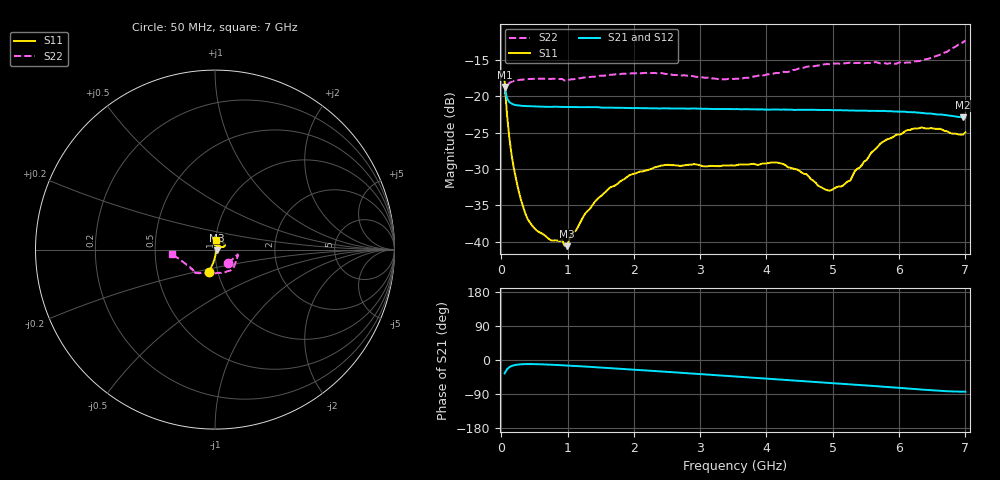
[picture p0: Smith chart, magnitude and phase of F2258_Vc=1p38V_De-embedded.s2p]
! Integrated Device Technology
! Corporate Headquarters
! 6024 Silver Creek Valley Road
! San Jose, CA 95138  USA
! Phone:  1-408-284-8200
! Toll Free:  1-800-223-1366
! Webpage:  http://www.idt.com/
! Timing and RF Division
! 515 Groton Road, Suite 102
! Westford, MA 01886-6024
! Device:  F2258
! Description: Voltage Variable RF Attenuator
! Frequency:  50.0 -  6000.00 MHz
! Package:  3x3 mm Thin QFN Plastic Package: 16 pin
! Ports:  2 RF, 2 DC
!  Pin  1  = NC
!  Pin  2  = NC
!  Pin  3  = RF2  = Port 2
!  Pin  4  = GND
!  Pin  5  = Vdd
!  Pin  6  = NC
!  Pin  7  = VCTRL
!  Pin  8  = NC
!  Pin  9  = GND
!  Pin 10  = RF1  = Port 1
!  Pin 11  = NC
!  Pin 12  = NC
!  Pin 13  = NC
!  Pin 14  = NC
!  Pin 15  = NC
!  Pin 16  = NC
! Vcntrl:  1.380 Volts
! Vdd:  +3.300 Volts
! Current:  1.166 mA
! Data:  The device was measured on a the F2258 evaluation board which has
!  individual transmission lines to the RF pins.  Data was collected
!  using a calibrated network analyzer.  The evaluation board was
!  de-embedded using a TRL calibration technique.
!  The reference plane is the edge of the package pin.
! Misc:  SN 10
!  Action Tracker AT0285
! Date Measured:  2014-12-10
! Date:  2016-01-13  MJV
! Note:
!  Integrated Device Technology supplies this data as a sample of measured
!  data at the package pin for this product.  Your particular data for this
!  product may vary.
!  Data was taken at 25 degrees C.
!  Integrated Device Technology reserves the right to change this data at anytime.
!Freq_(GHz)  S11M_(dB)  S11P_(deg)  S21M_(dB)  S21P_(deg)  S12M_(dB)  S12P_(deg)  S22M_(dB)  S22P_(deg)
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# GHz S dB R 50
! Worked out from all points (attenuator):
!   201 points, 50 MHz to 7 GHz, reference 50 ohm
!   highest |S21| = -18.72 dB at 50 MHz (marker M1); lowest = -22.9 dB at 6.965 GHz (marker M2)
!   lowest |S11| = -40.6 dB at 988.2 MHz (marker M3), VSWR 1.02, Z = 50.9 - j0.398 ohm
!   |S11| at or under -10 dB: start of sweep to end of sweep
!   |S22| runs from -19.7 to -12.3 dB; largest |S21 - S12| = 0.0006
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0.05  -17.93 -105.0  -18.72 -35.4  -18.73 -35.5  -19.68 -45.6
0.08475  -22.40 -97.9  -20.26 -24.7  -20.26 -24.7  -18.67 -22.8
0.15425  -28.01 -89.9  -21.01 -15.9  -21.03 -15.9  -18.01 -14.2
0.2585  -32.89 -79.7  -21.26 -11.9  -21.28 -11.9  -17.78 -12.0
0.36275  -36.12 -68.6  -21.35 -10.8  -21.36 -10.8  -17.67 -12.8
0.5365  -38.46 -49.0  -21.41 -11.0  -21.43 -11.0  -17.59 -15.5
0.98825  -40.60 -24.8  -21.48 -14.5  -21.50 -14.5  -17.80 -25.9
1.05775  -38.96 -16.3  -21.48 -15.2  -21.52 -15.2  -17.68 -27.3
1.2315  -36.65 -5.0  -21.49 -17.0  -21.50 -17.0  -17.45 -31.0
1.6485  -32.50 6.2  -21.57 -21.6  -21.59 -21.6  -17.06 -39.4
1.9265  -30.89 15.1  -21.62 -24.7  -21.64 -24.7  -16.89 -44.8
2.37825  -29.61 26.8  -21.69 -29.8  -21.70 -29.8  -16.83 -54.0
3.525  -29.50 79.8  -21.77 -43.4  -21.78 -43.4  -17.62 -91.2
4.18525  -29.16 101.0  -21.83 -51.3  -21.82 -51.4  -16.81 -114.6
4.7065  -31.61 89.7  -21.87 -57.6  -21.84 -57.7  -15.90 -125.5
4.94975  -32.98 67.7  -21.92 -60.5  -21.89 -60.6  -15.59 -128.1
5.15825  -32.24 45.9  -21.94 -63.1  -21.91 -63.2  -15.49 -130.2
5.57525  -27.82 20.3  -22.01 -68.1  -21.97 -68.2  -15.45 -134.2
5.85325  -25.84 18.7  -22.06 -71.7  -22.03 -71.8  -15.49 -138.2
6.33975  -24.27 26.9  -22.30 -78.1  -22.26 -78.2  -15.10 -150.4
6.96525  -25.27 78.6  -22.91 -83.7  -22.91 -83.7  -12.58 -173.1
7  -24.97 83.7  -22.91 -83.8  -22.91 -83.8  -12.34 -174.5
